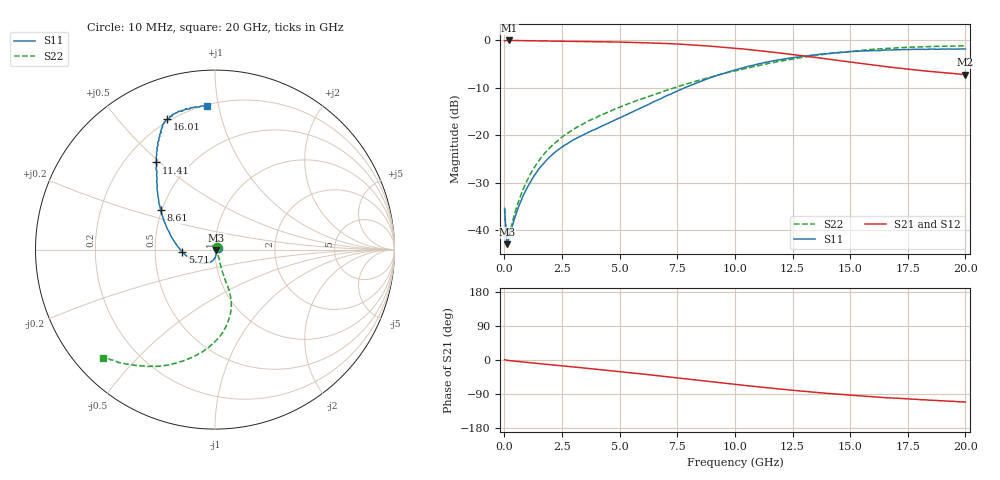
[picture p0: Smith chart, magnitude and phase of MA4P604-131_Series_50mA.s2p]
! AWR Design Environment (9226) Thu Aug 19 15:08:55 2021
! Document = '50mA'
! nPorts: 2, nXvals: 201
# GHz S DB R 50
!Freq DBS11 AngS11 DBS21 AngS21 DBS12 AngS12 DBS22 AngS22
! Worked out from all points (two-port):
!   201 points, 10 MHz to 20 GHz, reference 50 ohm
!   highest |S21| = -0.12 dB at 210 MHz (marker M1); lowest = -7.3 dB at 20 GHz (marker M2)
!   |S21| within 3 dB of the highest: start of sweep to 12.57 GHz
!   lowest |S11| = -42.9 dB at 110 MHz (marker M3), VSWR 1.01, Z = 50.7 - j0.195 ohm
!   |S11| at or under -10 dB: start of sweep to 7.84 GHz
!   |S22| runs from -43.3 to -1.2 dB; largest |S21 - S12| = 0.028
!   S11 on the Smith chart (normalised r, x): 10 MHz: 1.03, +0.01; 5.71 GHz: 0.69, -0.02; 8.61 GHz: 0.49, +0.25; 11.41 GHz: 0.33, +0.49; 16.01 GHz: 0.19, +0.68; 20 GHz: 0.20, +0.92
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0.01  -35.66 24.3  -0.18 0.8  -0.15 0.7  -35.21 49.9
0.11  -42.94 -15.6  -0.12 -0.7  -0.10 -0.7  -43.31 -17.1
0.21  -41.40 -31.3  -0.12 -1.5  -0.10 -1.4  -41.00 -29.0
0.41  -37.99 -50.7  -0.13 -2.8  -0.11 -2.7  -37.13 -46.9
0.71  -33.94 -66.9  -0.15 -4.7  -0.13 -4.6  -32.65 -56.5
1.11  -29.97 -79.9  -0.18 -7.2  -0.16 -7.0  -28.31 -62.3
1.41  -27.72 -87.2  -0.20 -9.0  -0.18 -8.7  -25.95 -64.9
1.81  -25.35 -96.1  -0.23 -11.3  -0.21 -11.0  -23.46 -67.4
2.21  -23.54 -104.9  -0.25 -13.7  -0.24 -13.3  -21.58 -69.3
3.41  -19.96 -129.8  -0.33 -20.8  -0.31 -20.3  -17.65 -71.5
4.71  -17.00 -156.5  -0.43 -28.7  -0.41 -28.1  -14.69 -71.4
5.71  -14.76 -175.9  -0.54 -35.1  -0.52 -34.3  -12.80 -70.8
6.71  -12.51 167.2  -0.69 -41.8  -0.67 -40.8  -11.13 -71.8
8.61  -8.52 143.9  -1.20 -54.7  -1.16 -53.4  -8.25 -78.1
10.01  -6.32 131.7  -1.74 -64.4  -1.68 -62.7  -6.52 -85.6
11.41  -4.64 124.1  -2.44 -73.3  -2.34 -71.7  -4.99 -95.8
13.41  -3.17 116.8  -3.63 -84.7  -3.47 -83.5  -3.33 -110.6
16.01  -2.24 110.1  -5.27 -97.2  -5.18 -96.4  -1.97 -126.5
16.71  -2.15 108.1  -5.70 -100.1  -5.65 -99.2  -1.74 -129.4
18.21  -1.98 103.5  -6.50 -104.8  -6.57 -104.6  -1.44 -134.0
19.51  -1.94 97.1  -7.06 -109.1  -7.24 -108.5  -1.29 -135.7
20  -1.89 93.3  -7.29 -111.2  -7.53 -110.0  -1.22 -136.1
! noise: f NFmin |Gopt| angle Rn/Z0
0.01  0  1  0  2e-20
2.21  0  1  0  2e-20
4.41  0  1  0  2e-20
6.61  0  1  0  2e-20
8.81  0  1  0  2e-20
11.11  0  1  0  2e-20
13.31  0  1  0  2e-20
15.51  0  1  0  2e-20
17.71  0  1  0  2e-20
20  0  1  0  2e-20
